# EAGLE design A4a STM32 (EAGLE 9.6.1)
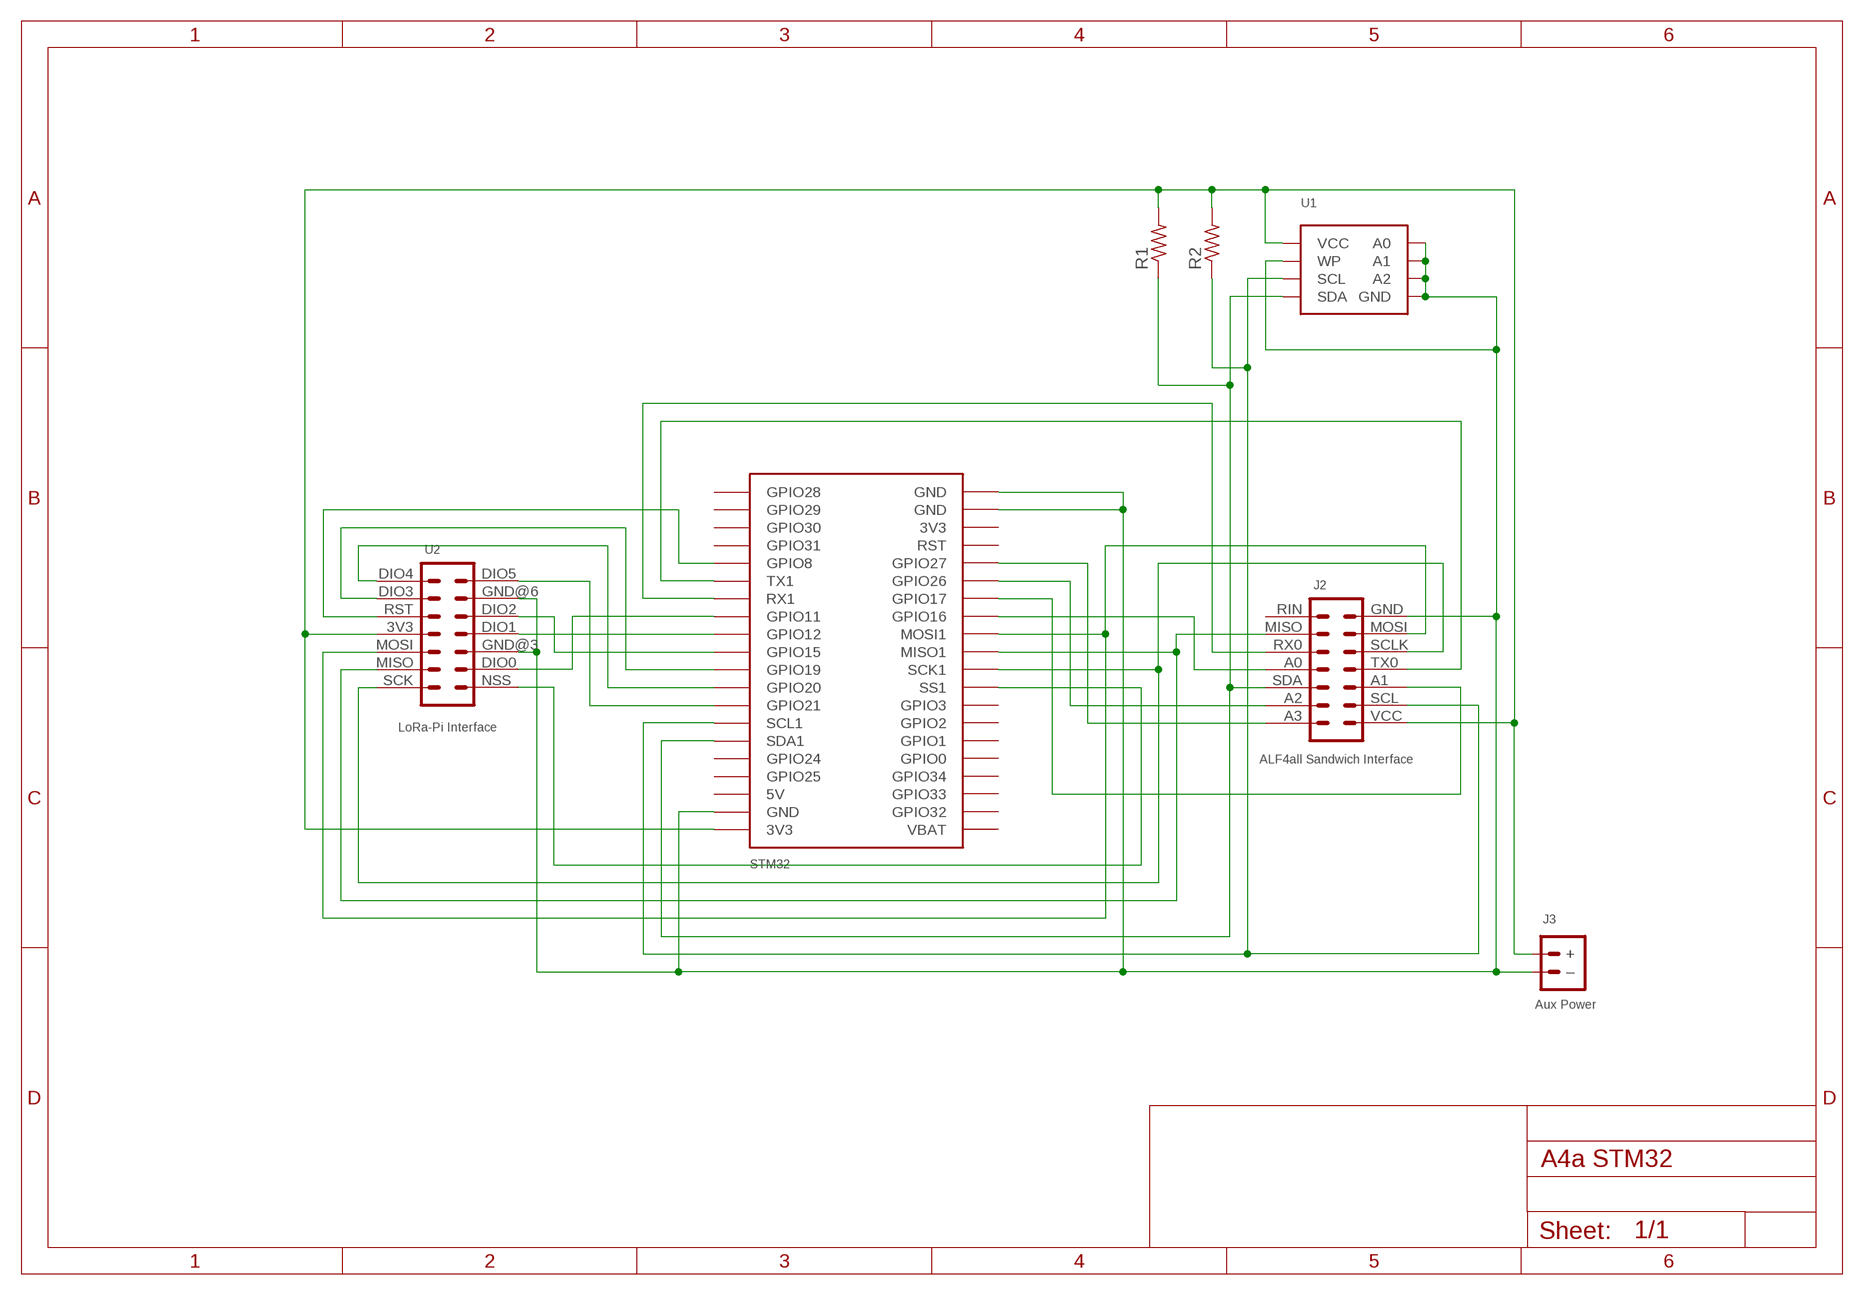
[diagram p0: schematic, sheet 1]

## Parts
J1  STM32  [STM32]
J2  ALF4all Sandwich Interface  HEADER-3X5-ALF4ALL-STM32-INTERCONNECT  [CONN_3X5-ALF4ALL-STM32-INTERCONNECT]
J3  Aux Power  JST-PH2.0-2-MALE-HORIZONTALJST-PTH-2  [JST-PH2.0-2-HORIZONTAL]
R1  RESISTORR0805  [R0805]
R2  RESISTORR0805  [R0805]
U1  AT24CXX-EEPROM-VIA-4  [SOP-8-WITH-VIA-4]
U2  LoRa-Pi Interface  RFM95W-PI-HEADER  [RFM95W-PI]

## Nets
GND: J1.GND@19(GND) J1.GND@20(GND) J1.GND@39(GND) J2.GND J3.-(–) U1.P$1(A0) U1.P$2(A1) U1.P$3(A2) U1.P$4(GND) U1.P$4@VIA(GND) U1.P$7(WP) U2.GND@3 U2.GND@6
N$1: J1.GPIO10(RX1) J2.RX0
N$2: J1.GPIO26 J2.A2
N$3: J1.GPIO22(SCL1) J2.SCL R2.1 U1.P$6(SCL)
N$4: J1.GPIO23(SDA1) J2.SDA R1.1 U1.P$5(SDA)
N$5: J1.GPIO16 J2.A0
N$6: J1.GPIO9(TX1) J2.TX0
N$7: J1.GPIO7(MOSI1) J2.MOSI U2.MOSI
N$8: J1.GPIO6(MISO1) J2.MISO U2.MISO
N$9: J1.GPIO27 J2.A3
N$11: J1.GPIO5(SCK1) J2.SCLK U2.SCK
N$12: J1.GPIO4(SS1) U2.NSS
N$13: J1.GPIO11 U2.DIO0
N$14: J1.GPIO12 U2.DIO1
N$15: J1.GPIO15 U2.DIO2
N$16: J1.GPIO19 U2.DIO3
N$17: J1.GPIO20 U2.DIO4
N$18: J1.GPIO21 U2.DIO5
N$19: J1.GPIO8 U2.RST
N$21: J1.GPIO17 J2.A1
VCC: J1.3V3@40(3V3) J2.VCC J3.+ R1.2 R2.2 U1.P$8(VCC) U2.3V3
Unconnected: J1.3V3@18(3V3) J1.5V@38(5V) J1.GPIO0 J1.GPIO1 J1.GPIO2 J1.GPIO3 J1.GPIO24 J1.GPIO25 J1.GPIO28 J1.GPIO29 J1.GPIO30 J1.GPIO31 J1.GPIO32 J1.GPIO33 J1.GPIO34 J1.RST J1.VBAT J2.RIN

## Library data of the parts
J1 = digitalconcepts:STM32: STM32 Development Board
J2 = digitalconcepts:HEADER-3X5-ALF4ALL-STM32-INTERCONNECT: ALF4all 'Sandwich' STM32 Interconnect 3x5 Pin Header Header soldered to top side of PCB
J3 = digitalconcepts:JST-PH2.0-2-MALE-HORIZONTAL: Multi connection point. Often used as Generic Header-pin footprint for 0.1 inch spaced/style header connections; PROD_ID: CONN-09863; SKU: PRT-09914
R1 R2 = digitalconcepts:RESISTOR: Resistor; SPICEPREFIX: R
U1 = digitalconcepts:AT24CXX-EEPROM-VIA-4: AT24Cxx EEPROM SOP-8
U2 = digitalconcepts:RFM95W-PI-HEADER: RFM95W LoRa Wireless Transceiver Raspberry Pi Daughter Board

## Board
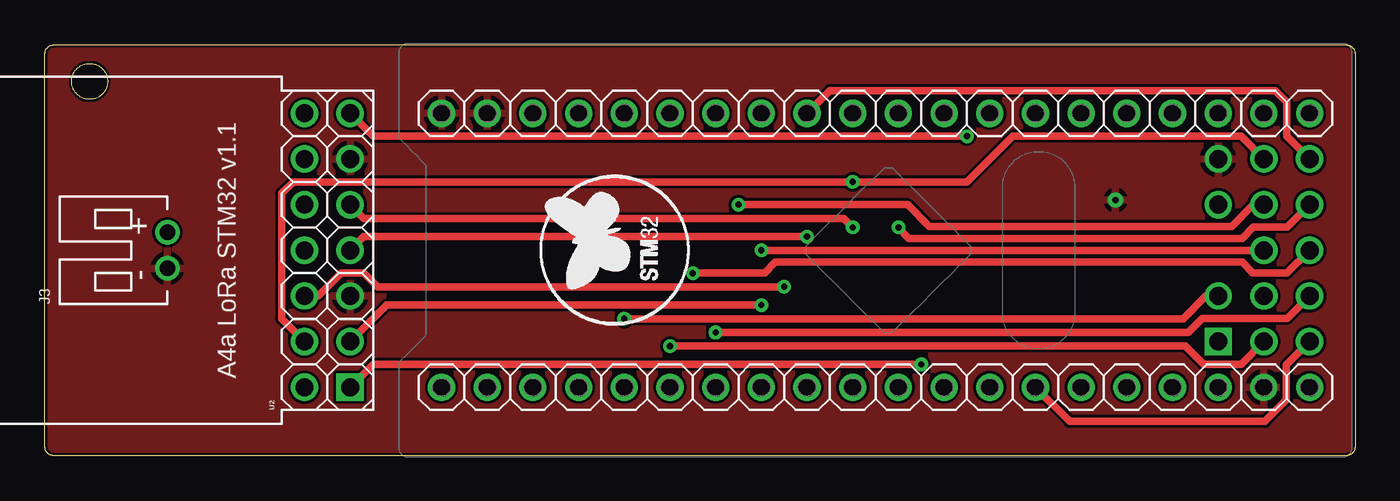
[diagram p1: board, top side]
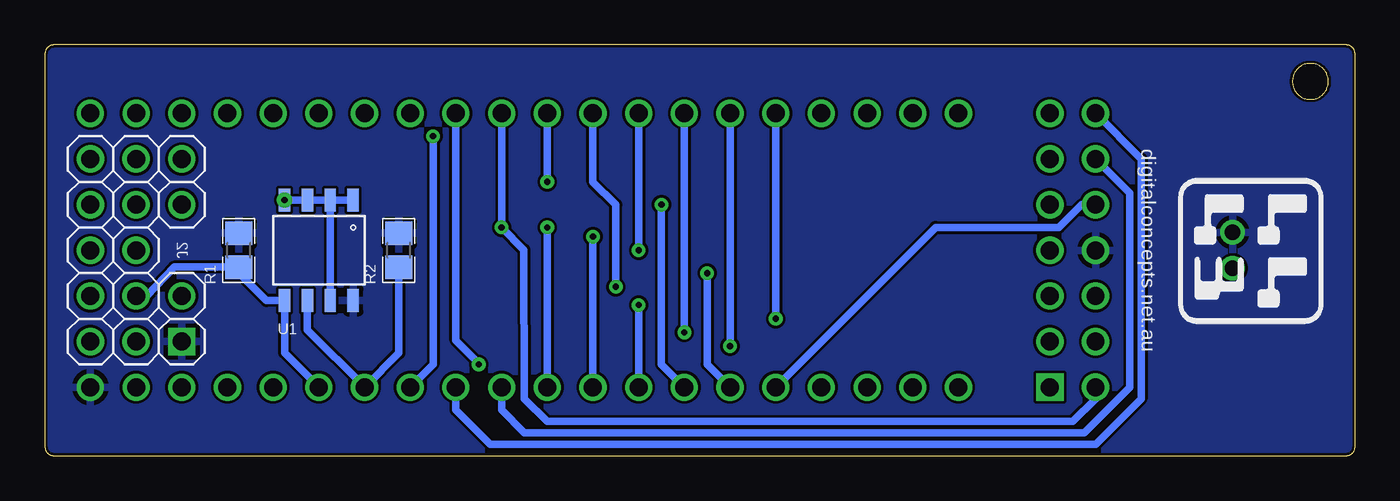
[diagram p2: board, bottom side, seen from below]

Size 72.84 x 22.86 mm. Coordinates in mm from the lower left corner, seen from the top.
Outline: 180 segments
Copper layers (1*16): Top 0.035mm / dielectric 1.5mm / Bottom 0.035mm
Design rules "default *": minimum track width 6mil, minimum drill 0.35mm, track to track 6mil, track to pad 6mil, pad to pad 6mil, via to via 6mil, smd to smd 6mil, copper to edge 6mil, drill to drill 6mil, minimum pad ring 10mil, minimum via ring 8mil, stop-mask expansion 4mil, vias tented up to drill 0mil, thermal gap 10mil

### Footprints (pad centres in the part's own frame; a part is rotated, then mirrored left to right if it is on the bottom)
STM32 = drill 1: 3V3@18 0,43.18; 3V3@40 -15.24,0; 5V@38 -15.24,5.08; GND@19 0,45.72; GND@20 0,48.26; GND@39 -15.24,2.54; GPIO0 0,10.16; GPIO1 0,12.7; GPIO2 0,15.24; GPIO3 0,17.78; GPIO4 0,20.32; GPIO5 0,22.86; GPIO6 0,25.4; GPIO7 0,27.94; GPIO8 -15.24,38.1; GPIO9 -15.24,35.56; GPIO10 -15.24,33.02; GPIO11 -15.24,30.48; GPIO12 -15.24,27.94; GPIO15 -15.24,25.4; GPIO16 0,30.48; GPIO17 0,33.02; GPIO19 -15.24,22.86; GPIO20 -15.24,20.32; GPIO21 -15.24,17.78; GPIO22 -15.24,15.24; GPIO23 -15.24,12.7; GPIO24 -15.24,10.16; GPIO25 -15.24,7.62; GPIO26 0,35.56; GPIO27 0,38.1; GPIO28 -15.24,48.26; GPIO29 -15.24,45.72; GPIO30 -15.24,43.18; GPIO31 -15.24,40.64; GPIO32 0,2.54; GPIO33 0,5.08; GPIO34 0,7.62; RST 0,40.64; VBAT 0,0
CONN_3X5-ALF4ALL-STM32-INTERCONNECT = drill 1 pad 1.524: A0 5.08,-2.54; A1 2.54,-5.08; A2 0,-2.54; A3 2.54,0; GND 10.16,0; MISO 10.16,-2.54; MOSI 10.16,-5.08; RIN 7.62,0; RX0 7.62,-2.54; SCL 0,-5.08; SCLK 7.62,-5.08; SDA 2.54,-2.54; TX0 5.08,-5.08 | drill 1 pad 1.524 square: VCC 0,0
JST-PH2.0-2-HORIZONTAL = drill 0.85: + 1,0; - -1,0
R0805 = smd 1.3 x 1.5: 1 -0.95,0; 2 0.95,0
SOP-8-WITH-VIA-4 = smd 0.635 x 1.27: P$1 -1.905,-2.794; P$2 -0.635,-2.794; P$3 0.635,-2.794; P$4 1.905,-2.794; P$5 1.905,2.794; P$6 0.635,2.794; P$7 -0.635,2.794; P$8 -1.905,2.794 | drill 0.35 pad 0.61: P$4@VIA 1.905,-2.794
RFM95W-PI = drill 1 pad 1.524: 3V3 7.62,2.54; DIO0 2.54,0; DIO1 7.62,0; DIO2 10.16,0; DIO3 12.7,2.54; DIO4 15.24,2.54; DIO5 15.24,0; GND@3 5.08,0; GND@6 12.7,0; MISO 2.54,2.54; MOSI 5.08,2.54; RST 10.16,2.54; SCK 0,2.54 | drill 1 pad 1.524 square: NSS 0,0

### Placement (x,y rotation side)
J1  70.31,19.05 90 top
J2  65.23,6.35 90 top
J3  6.81,11.43 90 top
R1  62.05,11.43 90 bottom
R2  53.16,11.43 90 bottom
U1  57.61,11.43 180 bottom
U2  16.97,3.81 90 top

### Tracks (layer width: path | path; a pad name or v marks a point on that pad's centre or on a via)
GND
  Bottom 0.406: U1.P$4@VIA U1.P$3 U1.P$2 | U1.P$2 U1.P$1 | U1.P$2 U1.P$7
  pour Top (rank 3): -2.08,25.4 75.39,25.4 75.39,-2.54 -2.08,-2.54
N$1  (via drill 0.35)
  Top 0.406: J2.RX0 67.19,13.97 65.99,12.75 49.15,12.75 47.96,13.97 v38.56,13.97
  Bottom 0.406: J1.GPIO10 38.56,5.08 v38.56,13.97
N$2  (via drill 0.35)
  Top 0.406: J2.A2 66.5,5.08 64.42,5.08 63.4,6.1 v34.75,6.1
  Bottom 0.406: J1.GPIO26 v34.75,6.1
N$3
  Top 0.406: J1.GPIO22 56.97,1.9 67.82,1.9 69.01,3.1 69.01,5.05 J2.SCL
  Bottom 0.406: R2.1 53.16,5.71 J1.GPIO22 55.07,3.82 58.24,7 U1.P$6
N$4
  Bottom 0.406: J2.SDA 67.19,8.89 65.65,10.49 62.17,10.49 62.16,10.48 R1.1 62.05,10.16 60.53,8.64 U1.P$5 59.51,5.73 57.61,3.82 J1.GPIO23
N$5  (via drill 0.35)
  Top 0.406: J2.A0 v39.83,11.43
  Bottom 0.406: J1.GPIO16 v39.83,11.43
N$6  (via drill 0.35)
  Top 0.406: J2.TX0 69.04,10.16 67.16,10.16 66.58,10.77 40.59,10.77 40.01,10.16 v36.02,10.16
  Bottom 0.406: v36.02,10.16 36.02,5.08 J1.GPIO9
N$7  (via drill 0.35)
  Top 0.406: v41.1,9.4 18.49,9.4 17.73,10.16 16.46,10.16 15.19,8.89 U2.MOSI | J2.MOSI 69.04,17.78 69.04,19.68 68.4,20.32 43.64,20.32 J1.GPIO7
  Bottom 0.406: J1.GPIO7 42.37,15.24 41.1,13.97 v41.1,9.4
N$8  (via drill 0.35)
  Top 0.406: J2.MISO 66.5,17.78 53.8,17.78 51.26,15.24 v44.91,15.24 13.79,15.24 13.16,14.6 13.16,7.62 U2.MISO
  Bottom 0.406: v44.91,15.24 J1.GPIO6
N$9  (via drill 0.35)
  Top 0.406: J2.A3 64.54,8.89 63.27,7.62 v32.21,7.62
  Bottom 0.406: J1.GPIO27 v32.21,7.62
N$11  (via drill 0.35)
  Top 0.406: J2.SCLK 69.06,12.72 67.19,12.72 66.58,12.09 48.03,12.09 v47.45,12.7
  Bottom 0.406: J1.GPIO5 v47.45,12.7 46.2,11.45 46.18,3.17 44.91,1.9 15.7,1.9 14.43,3.17 U2.SCK
N$12  (via drill 0.35)
  Top 0.406: U2.NSS 18.24,5.08 v48.72,5.08
  Bottom 0.406: J1.GPIO4 49.99,6.42 48.72,5.13 v48.72,5.08
N$13  (via drill 0.35)
  Top 0.406: v39.83,8.38 19,8.38 U2.DIO0
  Bottom 0.406: v39.83,8.38 J1.GPIO11
N$14  (via drill 0.35)
  Top 0.406: U2.DIO1 17.73,12.19 v42.37,12.19
  Bottom 0.406: v42.37,12.19 J1.GPIO12
N$15  (via drill 0.35)
  Top 0.406: U2.DIO2 17.73,13.21 44.4,13.21 v44.91,12.7
  Bottom 0.406: v44.91,12.7 J1.GPIO15
N$16
  Bottom 0.406: U2.DIO3 12.52,14.6 12.52,3.81 15.06,1.27 46.18,1.27 47.45,2.54 J1.GPIO19
N$17
  Bottom 0.406: U2.DIO4 11.89,16.51 11.89,3.17 14.43,0.63 48.08,0.63 49.99,2.54 J1.GPIO20
N$18  (via drill 0.35)
  Top 0.406: U2.DIO5 18.24,17.78 v51.26,17.78
  Bottom 0.406: v51.26,17.78 51.26,5.08 J1.GPIO21
N$19
  Bottom 0.406: U2.RST 15.19,13.97 16.46,12.7 23.32,12.7 J1.GPIO8
N$21  (via drill 0.35)
  Top 0.406: J2.A1 69.06,7.64 64.34,7.64 63.55,6.86 v37.29,6.86
  Bottom 0.406: J1.GPIO17 v37.29,6.86
VCC
  pour Bottom (rank 3): -0.81,24.13 74.12,24.13 74.12,-1.27 -0.81,-1.27

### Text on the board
tPlace: A4a LoRa STM32 v1.1
bPlace: digitalconcepts.net.au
